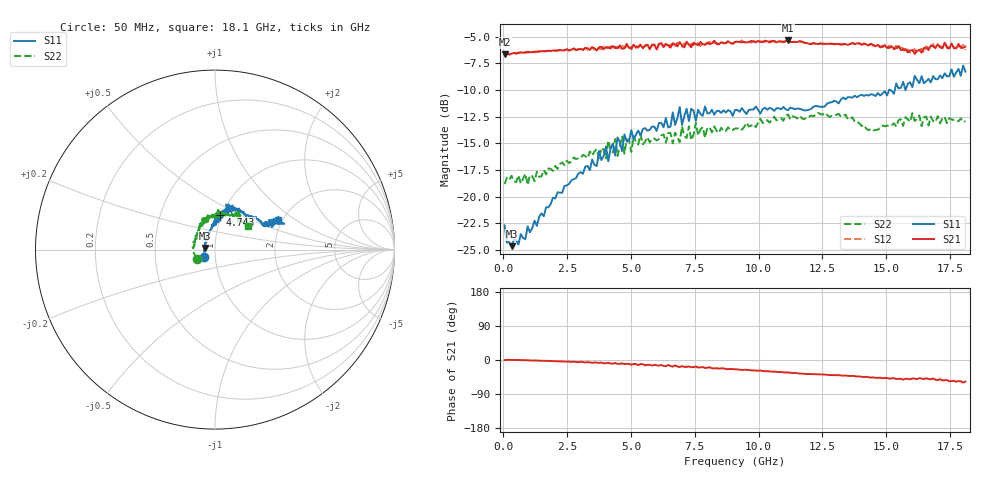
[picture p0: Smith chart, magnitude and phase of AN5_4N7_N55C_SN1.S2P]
! Network Analyzer HP8720D.06.14 Serial No. US36140669
!  5 Jul 2005  06:51:53
! Frequency  S11  S21  S12  S22
# HZ  S  DB R 50
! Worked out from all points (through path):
!   201 points, 50 MHz to 18.1 GHz, reference 50 ohm
!   highest |S21| = -5.34 dB at 11.15 GHz (marker M1); lowest = -6.6 dB at 50 MHz (marker M2)
!   group delay of S21, straight-line fit = 9.4 ps
!   lowest |S11| = -24.6 dB at 320.8 MHz (marker M3), VSWR 1.12, Z = 44.5 + j0.86 ohm
!   |S11| at or under -10 dB: start of sweep to 15.11 GHz; 15.16 GHz to 15.34 GHz (172.9 MHz wide, 1.13 % of centre); 15.75065 GHz to 15.75717 GHz (6.521 MHz wide, 0.0414 % of centre)
!   |S22| runs from -18.9 to -12.1 dB; largest |S21 - S12| = 0.029
!   S11 on the Smith chart (normalised r, x): 50 MHz: 0.88, -0.08; 4.743 GHz: 0.98, +0.40; 18.1 GHz: 1.89, +0.73
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5e7  -22.70 -144.6  -6.65 -0.3  -6.68 -0.0  -18.82 -154.1
3.2075e8  -24.65 170.5  -6.59 0.1  -6.59 -0.1  -18.04 174.1
9.525e8  -22.79 137.5  -6.40 -0.7  -6.49 -0.3  -18.89 157.4
3.1185e9  -17.85 96.4  -6.22 -5.3  -6.24 -5.9  -16.09 123.6
4.021e9  -15.29 88.6  -5.96 -8.7  -6.12 -7.2  -16.42 114.0
4.11125e9  -16.69 87.9  -6.02 -7.1  -6.01 -9.1  -14.73 112.2
4.29175e9  -15.03 91.0  -5.85 -9.6  -6.22 -9.2  -15.86 105.6
4.382e9  -16.16 84.6  -6.04 -7.9  -5.95 -9.7  -14.60 111.9
4.47225e9  -14.44 79.4  -6.08 -10.1  -5.95 -8.0  -16.19 115.4
4.65275e9  -15.72 79.3  -6.13 -8.8  -5.83 -10.0  -14.37 113.0
4.743e9  -14.16 81.6  -6.07 -10.8  -6.06 -9.3  -15.96 108.8
5.104e9  -14.64 82.8  -5.74 -10.6  -5.79 -11.7  -14.29 102.7
6.09675e9  -13.09 74.5  -5.72 -15.0  -5.62 -14.3  -14.60 95.8
6.7285e9  -13.27 77.4  -5.70 -14.3  -6.01 -15.7  -13.99 87.0
6.909e9  -11.59 73.1  -5.50 -18.6  -5.69 -16.3  -14.90 85.4
6.99925e9  -13.27 73.2  -5.81 -16.2  -5.93 -18.6  -13.39 85.3
7.17975e9  -11.75 76.3  -5.47 -18.2  -5.83 -16.8  -14.50 79.9
9.075e9  -11.87 64.4  -5.49 -24.4  -5.47 -24.3  -13.61 68.3
1.115075e10  -11.89 51.9  -5.34 -32.8  -5.37 -33.5  -12.28 57.7
1.21435e10  -11.57 46.4  -5.62 -37.2  -5.57 -37.0  -12.45 59.0
1.512175e10  -9.95 25.1  -6.06 -49.2  -5.82 -48.5  -13.38 47.5
1.81e10  -8.27 25.3  -5.92 -57.1  -6.24 -57.2  -12.92 34.9
